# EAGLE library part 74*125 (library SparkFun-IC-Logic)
Quad inverter with enable BUFF TRI-ST QD N-INV 14SOIC SparkFun Products Pocket AVR Programmer (PGM-09825) SparkFun Line Follower Array (SEN-13582)
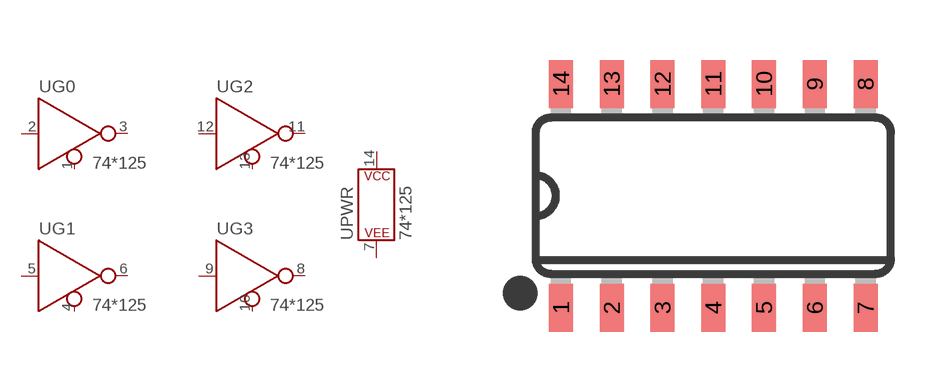
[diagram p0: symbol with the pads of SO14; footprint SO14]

Designator prefix U; gates G0=GATE_INVERTER_WITH_ENABLE G1=GATE_INVERTER_WITH_ENABLE G2=GATE_INVERTER_WITH_ENABLE G3=GATE_INVERTER_WITH_ENABLE PWR=POWER_CONSORT

## 74AC125DG (PROD_ID: IC-08880; VALUE: MC74AC125DG)  [SO14]
1  G0:!EN
2  G0:A
3  G0:Y
4  G1:!EN
5  G1:A
6  G1:Y
7  PWR:P$V-
8  G3:Y
9  G3:A
10  G3:!EN
11  G2:Y
12  G2:A
13  G2:!EN
14  PWR:P$V+

## Footprint SO14 (pad centres in mm)
smd 0.6 x 1.2: 1 -3.175,-2.8; 2 -1.905,-2.8; 3 -0.635,-2.8; 4 0.635,-2.8; 5 1.905,-2.8; 6 3.175,-2.8; 7 4.445,-2.8; 8 4.445,2.8; 9 3.175,2.8; 10 1.905,2.8; 11 0.635,2.8; 12 -0.635,2.8; 13 -1.905,2.8; 14 -3.175,2.8

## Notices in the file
Licensing: Creative Commons ShareAlike 4.0 International - https://creativecommons.org/licenses/by-sa/4.0
